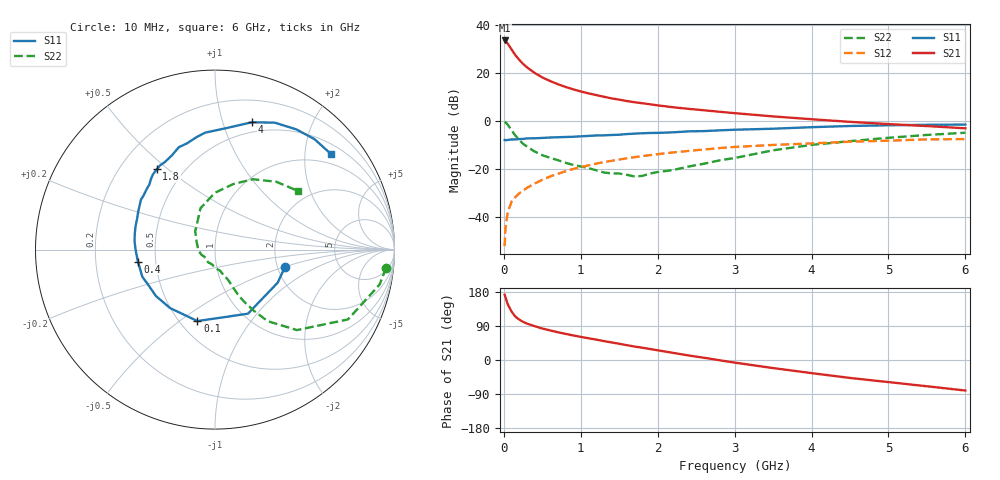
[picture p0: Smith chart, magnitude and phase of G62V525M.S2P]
! SIEMENS Small Signal Semiconductors
! BFG193
! Si NPN RF Bipolar Junction Transistor in SOT223
! VCE = 2.5 V  IC = 25 mA
! Common Emitter S-Parameters:  August  1996
# GHz  S  MA  R  50
!  f  S11  S21  S12  S22
! GHz  MAG  ANG  MAG  ANG  MAG  ANG  MAG  ANG
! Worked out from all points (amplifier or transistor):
!   36 points, 10 MHz to 6 GHz, reference 50 ohm
!   highest |S21| = 33.4 dB at 10 MHz (marker M1)
!   |S21| within 3 dB of that: start of sweep to 85.29 MHz
!   unconditionally stable (mu >= 1): 623.4 MHz to 2.552 GHz
!   at 250 MHz: K = 0.81, MSG = 26.3 dB, |S12| = -29.0 dB
!   at 1.4 GHz: K = 1.05, MAG = 11.6 dB, |S12| = -16.6 dB
!   at 6 GHz: K = 0.90, MSG = 2.2 dB, |S12| = -7.6 dB
!   S11 on the Smith chart (normalised r, x): 10 MHz: 2.20, -0.50; 100 MHz: 0.61, -0.58; 400 MHz: 0.40, -0.07; 1.8 GHz: 0.36, +0.46; 4 GHz: 0.40, +1.25; 6 GHz: 0.73, +2.59
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0.01  0.4017 -13.8  46.67 172.5  0.0025 87.2  0.9585 -6.1
0.02  0.395 -27.8  45.41 166.3  0.0057 79.5  0.9373 -12.0
0.05  0.4014 -62.8  40.26 147.4  0.0125 72.6  0.8368 -27.7
0.1  0.41 -103.8  30.43 127.8  0.021 62.6  0.6397 -44.5
0.15  0.4107 -127.4  23.11 114.5  0.0263 59.0  0.4941 -53.7
0.2  0.4187 -141.8  18.51 106.7  0.0312 59.9  0.4026 -57.6
0.25  0.4208 -152.4  15.25 100.7  0.0356 60.3  0.334 -60.7
0.3  0.4322 -159.5  12.93 96.1  0.0406 61.5  0.2926 -62.6
0.4  0.4346 -171.1  9.911 89.4  0.0498 62.5  0.2306 -64.7
0.5  0.4416 -179.3  7.982 83.1  0.0596 62.4  0.1936 -66.0
0.6  0.451 174.0  6.721 78.1  0.0698 62.3  0.1712 -67.9
0.7  0.4563 168.1  5.791 73.4  0.0793 61.1  0.1527 -70.9
0.9  0.4668 158.3  4.524 64.9  0.1001 58.4  0.1219 -76.1
1.1  0.4866 149.7  3.721 57.4  0.1191 55.6  0.1047 -87.9
1.4  0.5084 138.5  2.931 46.4  0.1477 49.8  0.0811 -109.3
1.8  0.5525 126.0  2.322 32.4  0.1853 41.6  0.072 -147.7
2.2  0.5776 114.5  1.916 18.8  0.221 32.4  0.0952 175.3
3.5  0.6866 83.0  1.236 -21.3  0.3161 1.6  0.2444 109.3
4  0.7383 73.9  1.081 -34.6  0.3398 -8.2  0.3167 90.1
4.5  0.7817 64.8  0.952 -47.4  0.3692 -18.3  0.3786 74.5
5.5  0.8282 48.0  0.779 -69.3  0.4125 -41.4  0.5095 47.9
6  0.837 39.7  0.7 -80.6  0.4175 -54.7  0.5663 35.2
